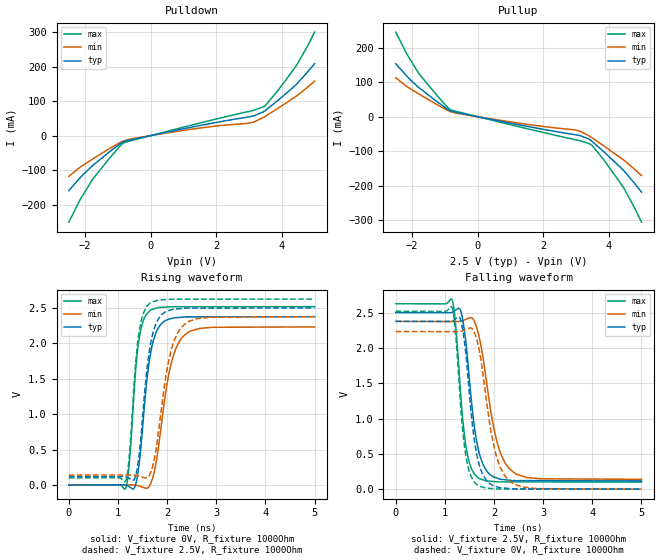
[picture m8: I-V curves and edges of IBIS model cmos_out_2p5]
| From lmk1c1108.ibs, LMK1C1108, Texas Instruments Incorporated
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[Model]   cmos_out_2p5
Model_type   Output
Polarity   Non-Inverting
Vmeas = 1.25
Vref = 0
Cref = 5pF
Rref = 100000
|   typ   min   max
C_comp   2.277pF   2.0763pF   2.5621pF
[Voltage Range]   2.5   2.375   2.625
[Temperature Range]   25   150   -40
[Pullup Reference]   2.5   2.375   2.625
[Pulldown Reference]   0   0   -0
[Power Clamp Reference]   2.5   2.375   2.625
[GND Clamp Reference]   0   0   0
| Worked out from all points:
|   slope of the pulldown table from 0 to 0.375 V, typ, clamps not added: 49.7 ohm
|   slope of the pullup table from 0 to 0.375 V, typ, clamps not added: 52.8 ohm
|   falling waveform, V_fixture 2.5V, R_fixture 1000Ohm: 20-80 % time 236ps typ, 334ps min, 187ps max; typ from 2.5 V to 0.116 V
|   rising waveform, V_fixture 0V, R_fixture 1000Ohm: 20-80 % time 216ps typ, 304ps min, 167ps max; typ from 0 V to 2.38 V
|   rising waveform, V_fixture 2.5V, R_fixture 1000Ohm: 20-80 % time 216ps typ, 300ps min, 168ps max; typ from 0.116 V to 2.5 V
|   falling waveform, V_fixture 0V, R_fixture 1000Ohm: 20-80 % time 225ps typ, 315ps min, 181ps max; typ from 2.38 V to 0 V
[Pulldown]
|   Voltage   I(typ)   I(min)   I(max)
-2.5V     -159.7mA   -118.4mA   -251.3mA
-2.185V   -125.4mA   -93.73mA   -191.3mA
-1.78V    -87.37mA   -68.48mA   -127.7mA
-872.5mV  -20.02mA   -17.06mA   -24.32mA
-617.5mV  -12.52mA   -10.01mA   -15.32mA
1.167V    22.99mA    17.49mA    28.54mA
3.027V    54.91mA    36.85mA    70.82mA
3.44V     69mA       52.84mA    83.64mA
3.897V    103.5mA    80.22mA    132.9mA
4.415V    145.9mA    112.7mA    199.1mA
4.812V    187.5mA    142.5mA    264.5mA
5V        208.9mA    158.1mA    300.4mA
[Pullup]
|   Voltage   I(typ)   I(min)   I(max)
-2.5V     153.6mA    113.1mA    245.3mA
-2.185V   120.3mA    89.3mA     186.1mA
-1.81V    85.75mA    66.93mA    127.8mA
-1.262V   45.33mA    36.03mA    64.18mA
-812.5mV  16.33mA    14.15mA    19.56mA
1.272V    -23.71mA   -18.81mA   -29.34mA
2.975V    -52.33mA   -38.64mA   -66.67mA
3.147V    -55.54mA   -42.85mA   -70.28mA
3.485V    -71.12mA   -60.84mA   -82.49mA
3.845V    -101.1mA   -84.37mA   -124.3mA
4.438V    -154.1mA   -124.3mA   -203.3mA
5V        -218.5mA   -170.6mA   -305.9mA
[Ramp]
R_load = 1000
|   typ   min   max
dV/dt_r   1.42593/2.16124e-10   1.33907/3.03532e-10   1.51114/1.66468e-10
dV/dt_f   1.43013/2.35883e-10   1.34128/3.33864e-10   1.51489/1.86762e-10
[Falling Waveform]
V_fixture = 2.5V
V_fixture_min = 2.375V
V_fixture_max = 2.625V
R_fixture = 1000Ohm
C_fixture = 0F
|   Time   V(typ)   V(min)   V(max)
0s        2.5V       2.375V     2.625V
1.143ns   2.504V     2.373V     2.688V
1.213ns   2.531V     2.373V     2.37V
1.307ns   2.549V     2.378V     1.487V
1.422ns   2.112V     2.402V     639mV
1.566ns   1.084V     2.414V     258.6mV
1.667ns   610mV      2.243V     166.4mV
2.024ns   165.2mV    774.4mV    106.2mV
2.313ns   126.4mV    290.4mV    102.9mV
5ns       116.4mV    139.5mV    100.2mV
[Rising Waveform]
V_fixture = 0V
V_fixture_min = 0V
V_fixture_max = 0V
R_fixture = 1000Ohm
C_fixture = 0F
|   Time   V(typ)   V(min)   V(max)
0s        11.5uV     10.11uV    12.29uV
1.161ns   -2.332mV   1.945mV    -40.83mV
1.237ns   -27.45mV   2.072mV    363.4mV
1.382ns   72.85mV    -4.482mV   1.788V
1.485ns   680.4mV    -26.14mV   2.255V
1.65ns    1.803V     -425uV     2.461V
1.775ns   2.153V     315.4mV    2.495V
2.051ns   2.343V     1.621V     2.516V
2.313ns   2.369V     2.089V     2.517V
5ns       2.377V     2.232V     2.519V
[Rising Waveform]
V_fixture = 2.5V
V_fixture_min = 2.375V
V_fixture_max = 2.625V
R_fixture = 1000Ohm
C_fixture = 0F
|   Time   V(typ)   V(min)   V(max)
0s        116.4mV    139.5mV    100.2mV
1.161ns   114.1mV    141.6mV    61.93mV
1.237ns   90.86mV    141.8mV    460.7mV
1.382ns   196.5mV    135.3mV    1.886V
1.485ns   833.6mV    114mV      2.353V
1.65ns    1.938V     155.1mV    2.565V
1.759ns   2.247V     434.7mV    2.597V
2.024ns   2.461V     1.726V     2.621V
2.287ns   2.491V     2.223V     2.623V
5ns       2.5V       2.375V     2.625V
[Falling Waveform]
|Gnd
V_fixture = 0V
V_fixture_min = 0V
V_fixture_max = 0V
R_fixture = 1000Ohm
C_fixture = 0F
|   Time   V(typ)   V(min)   V(max)
0s        2.377V     2.232V     2.519V
1.143ns   2.381V     2.23V      2.58V
1.213ns   2.408V     2.23V      2.245V
1.307ns   2.421V     2.234V     1.327V
1.422ns   1.951V     2.258V     497.9mV
1.566ns   880.4mV    2.262V     141.5mV
1.667ns   435.8mV    2.07V      58.13mV
1.98ns    52.52mV    665.5mV    7.624mV
2.262ns   12.17mV    154mV      2.397mV
5ns       11.5uV     10.11uV    12.29uV
